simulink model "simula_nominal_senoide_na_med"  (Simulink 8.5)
settings: Solver=ode45  StartTime=0.0  StopTime=tf  RelTol=1e-6
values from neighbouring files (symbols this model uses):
  denK = conv([1/3 1],[1 0.01])    [princi_JL_incerto_sem_prefilt_com_limit_ctrle.m]
  knom = r*kT/Ra/Jeq    [princi_JL_incerto_sem_prefilt_com_limit_ctrle.m]
  numK = 3.5*0.1*[1 0.1]    [princi_JL_incerto_sem_prefilt_com_limit_ctrle.m]
  pnom = feq/Jeq    [princi_JL_incerto_sem_prefilt_com_limit_ctrle.m]
  w0_med = wn    (= 10)    [princi_JL_incerto_sem_prefilt_com_limit_ctrle.m]

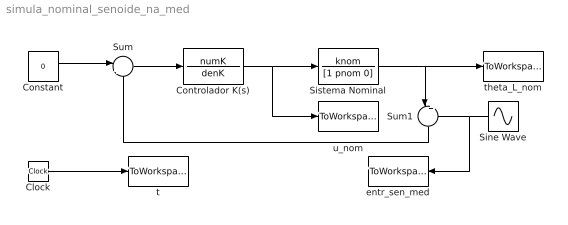
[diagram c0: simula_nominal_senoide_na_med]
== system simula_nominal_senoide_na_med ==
  Clock : Clock
  Constant : Constant  Value=0
  Controlador K(s) : TransferFcn  Numerator=numK  Denominator=denK
  Sine Wave : Sin  Frequency=w0_med  SampleTime=0
  Sistema Nominal : TransferFcn  Numerator=knom  Denominator=[1 pnom 0]
  Sum : Sum  Inputs=|+-
  Sum1 : Sum  Inputs=|++
  entr_sen_med : ToWorkspace  VariableName=entr_sen_med  SampleTime=-1
  t : ToWorkspace  VariableName=t_nom  SampleTime=-1
  theta_L_nom : ToWorkspace  VariableName=theta_L_nom  SampleTime=-1
  u_nom : ToWorkspace  VariableName=u_nom  SampleTime=-1
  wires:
  Sum/1 -> Controlador K(s)/1
  Clock/1 -> t/1
  Controlador K(s)/1 -> u_nom/1, Sistema Nominal/1
  Constant/1 -> Sum/1
  Sistema Nominal/1 -> theta_L_nom/1, Sum1/1
  Sine Wave/1 -> entr_sen_med/1, Sum1/2
  Sum1/1 -> Sum/2
